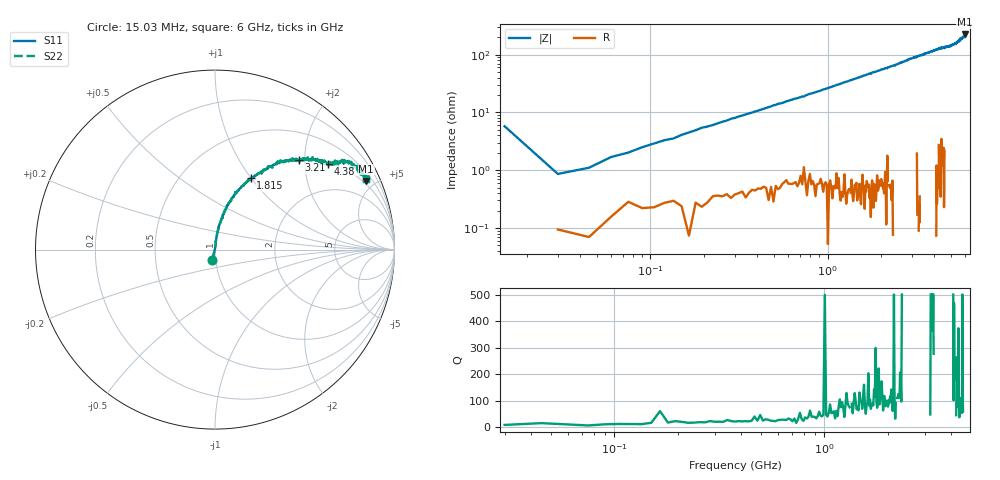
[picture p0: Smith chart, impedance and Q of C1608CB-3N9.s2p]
!	Network	Analyzer	HP8753E.07.74:	Oct	30	2002	Serial	No.	JP38451487
!	Hewlett-Packard
!	7	Sep	2009	9:30:22
!	Frequency	S11	S21	S12	S22
#	HZ	S	RI	R	50
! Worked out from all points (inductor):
!   400 points, 15.03 MHz to 6 GHz, reference 50 ohm
!   read as one part in series: L = 4.25 nH near 45.03 MHz
!   highest |Z| = 224 ohm at 5.955 GHz (marker M1)
!   S11 on the Smith chart (normalised r, x): 15.03 MHz: 0.96, -0.11; 1.815 GHz: 1.00, +0.99; 3.21 GHz: 1.00, +1.87; 4.38 GHz: 1.03, +2.62; 6 GHz: 0.75, +4.35
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1.502992e7  -0.015 -0.0561  1.02 0.0561  1.02 0.0561  -0.015 -0.0561
3.002985e7  0.00103 0.00856  0.999 -0.00856  0.999 -0.00856  0.00103 0.00856
4.502978e7  0.000638 0.011  0.999 -0.011  0.999 -0.011  0.000638 0.011
6.00297e7  0.0017 0.0168  0.998 -0.0168  0.998 -0.0168  0.0017 0.0168
1.200294e8  0.0036 0.0328  0.996 -0.0328  0.996 -0.0328  0.0036 0.0328
1.95029e8  0.00549 0.0539  0.995 -0.0539  0.995 -0.0539  0.00549 0.0539
2.850286e8  0.00947 0.0767  0.991 -0.0767  0.991 -0.0767  0.00947 0.0767
5.250274e8  0.0238 0.137  0.976 -0.137  0.976 -0.137  0.0238 0.137
1.020025e9  0.072 0.248  0.928 -0.248  0.928 -0.248  0.072 0.248
1.815021e9  0.199 0.397  0.801 -0.397  0.801 -0.397  0.199 0.397
2.01002e9  0.234 0.417  0.766 -0.417  0.766 -0.417  0.234 0.417
3.015015e9  0.432 0.508  0.568 -0.508  0.568 -0.508  0.432 0.508
3.210014e9  0.467 0.498  0.533 -0.498  0.533 -0.498  0.467 0.498
4.00501e9  0.596 0.498  0.404 -0.498  0.404 -0.498  0.596 0.498
4.380008e9  0.63 0.477  0.37 -0.477  0.37 -0.477  0.63 0.477
5.010005e9  0.685 0.488  0.315 -0.488  0.315 -0.488  0.685 0.488
5.385003e9  0.742 0.494  0.258 -0.494  0.258 -0.494  0.742 0.494
5.535002e9  0.752 0.453  0.248 -0.453  0.248 -0.453  0.752 0.453
5.565002e9  0.808 0.468  0.192 -0.468  0.192 -0.468  0.808 0.468
5.925e9  0.815 0.422  0.185 -0.422  0.185 -0.422  0.815 0.422
5.955e9  0.842 0.382  0.158 -0.382  0.158 -0.382  0.842 0.382
6e9  0.841 0.396  0.159 -0.396  0.159 -0.396  0.841 0.396
